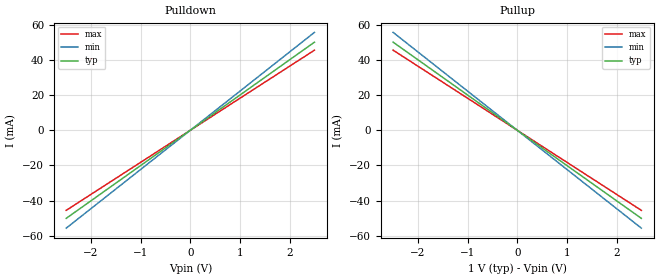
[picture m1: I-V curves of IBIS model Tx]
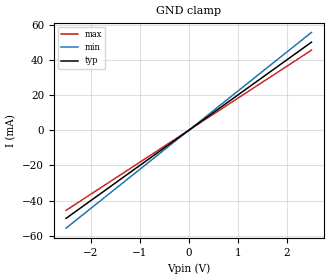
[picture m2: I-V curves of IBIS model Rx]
[IBIS Ver]   3.2
[Disclaimer] THIS IBIS MODEL HAS BEEN CREATED BY  SIGNAL
   INTEGRITY SOFTWARE
[File Name]  legacy.ibs
[File Rev]   1.0
[Date]   Tue Aug 28 14:09:44 EDT 2012
[Source]   Signal Integrity Software
   6 Clock Tower Place, Suite 250
   Maynard, MA 01754
   support@sisoft.com
   Auto-generated by "Create Default Model" dialog.
[Notes]   Note
[Copyright]  No Copyright
[Component]  legacy
[Manufacturer]  SiSoft
[Package]
R_pkg 0.001m   NA   NA
L_pkg 0.001nH  NA   NA
C_pkg 0.001pF  NA   NA
[Pin]  signal_name   model_name   R_pin  L_pin  C_pin
AW10 RX[0]_N Rx NA NA NA | Diff_Package pkg_{Corner}.mod pkg_{Corner} Length=0.01755
AV10 RX[0]_P Rx NA NA NA | Diff_Package pkg_{Corner}.mod pkg_{Corner} Length=0.01755
AW13 RX[1]_N Rx NA NA NA | Diff_Package pkg_{Corner}.mod pkg_{Corner} Length=0.01565
AV13 RX[1]_P Rx NA NA NA | Diff_Package pkg_{Corner}.mod pkg_{Corner} Length=0.01565
AW8 RX[10]_N Rx NA NA NA | Diff_Package pkg_{Corner}.mod pkg_{Corner} Length=0.01785
AV8 RX[10]_P Rx NA NA NA | Diff_Package pkg_{Corner}.mod pkg_{Corner} Length=0.01785
AR10 TX[0]_N Tx NA NA NA | Diff_Package pkg_{Corner}.mod pkg_{Corner} Length=0.01375
AP10 TX[0]_P Tx NA NA NA | Diff_Package pkg_{Corner}.mod pkg_{Corner} Length=0.01375
AR13 TX[1]_N Tx NA NA NA | Diff_Package pkg_{Corner}.mod pkg_{Corner} Length=0.01165
AP13 TX[1]_P Tx NA NA NA | Diff_Package pkg_{Corner}.mod pkg_{Corner} Length=0.01165
AR8 TX[10]_N Tx NA NA NA | Diff_Package pkg_{Corner}.mod pkg_{Corner} Length=0.01340
AP8 TX[10]_P Tx NA NA NA | Diff_Package pkg_{Corner}.mod pkg_{Corner} Length=0.01340
[Diff_Pin]  inv_pin  vdiff  tdelay_typ  tdelay_min  tdelay_max
AV10   AW10   0.1V   0.0ns   0.0ns   0.0ns
AV13   AW13   0.1V   0.0ns   0.0ns   0.0ns
AV8   AW8   0.1V   0.0ns   0.0ns   0.0ns
AP10   AR10   0.1V   0.0ns   0.0ns   0.0ns
AP13   AR13   0.1V   0.0ns   0.0ns   0.0ns
AP8   AR8   0.1V   0.0ns   0.0ns   0.0ns
| Models and submodels in the file (2): Tx (Output), Rx (Input)
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|   MODEL Tx
[Model] Tx
Model_type Output
C_comp 0.5p 0.5p 0.5p
Cref = 0
Vref = 0.5
Rref = 50
Vmeas = 0.5
[Temperature_Range] 25 100 0
[Voltage Range] 1.0 1.0 1.0
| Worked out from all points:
|   slope of the pulldown table from 0 to 0.15 V, typ, clamps not added: 50 ohm
|   slope of the pullup table from 0 to 0.15 V, typ, clamps not added: 50 ohm
| On-Die Tstonefile Tx_typ.s4p Tx_min.s4p Tx_max.s4p
| Diff_Package pkg_{Corner}.mod pkg_{Corner} Length=0.02
| Diff_Package_Coupled pkg_cpl_{Corner}.mod pkg_cpl_{Corner} Length=0.02
[Pulldown]
-2.5V     -50mA      -55.56mA   -45.45mA
0V        0A         0A         0A
2.5V      50mA       55.56mA    45.45mA
[Pullup]
-2.5V     50mA       55.56mA    45.45mA
0V        0A         0A         0A
2.5V      -50mA      -55.56mA   -45.45mA
[Ramp]
dV/dt_r .3/60p .3/60p .3/60p
dV/dt_f .3/60p .3/60p .3/60p
|   MODEL Rx
[Model] Rx
Model_type Input
C_comp 0.5p 0.5p 0.5p
Vinh = 0.55
Vinl = 0.45
[Temperature_Range] 25 100 0
[Voltage Range] 1.0 1.0 1.0
| On-Die Tstonefile Rx_typ.s4p Rx_min.s4p Rx_max.s4p
| Diff_Package pkg_{Corner}.mod pkg_{Corner} Length=0.01
| Diff_Package_Coupled pkg_cpl_{Corner}.mod pkg_cpl_{Corner} Length=0.01
[GND Clamp]
-2.5V     -50mA      -55.56mA   -45.45mA
0V        0A         0A         0A
2.5V      50mA       55.56mA    45.45mA
